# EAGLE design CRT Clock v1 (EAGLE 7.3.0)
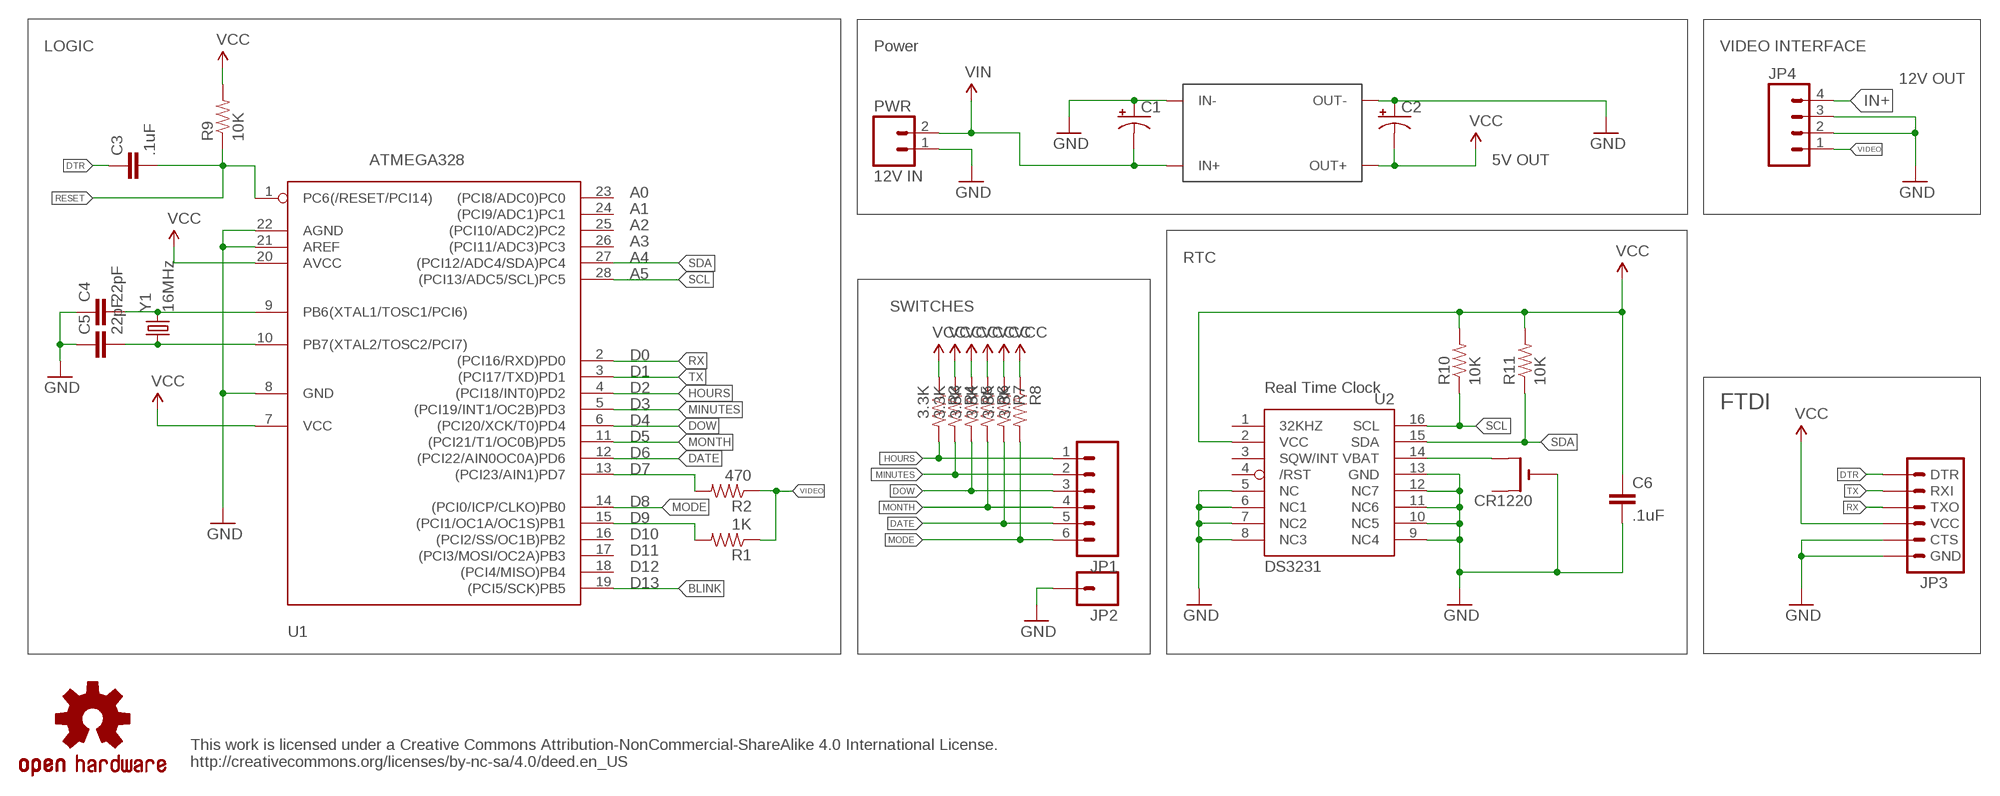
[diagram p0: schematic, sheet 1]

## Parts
C1  CAP_POLPTH2  [CPOL-RADIAL-10UF-25V]
C2  CAP_POLPTH2  [CPOL-RADIAL-10UF-25V]
C3  .1uF  CAPEZ  [CAP-PTH-SMALLEZ]
C4  22pF  CAPEZ  [CAP-PTH-SMALLEZ]
C5  22pF  CAPEZ  [CAP-PTH-SMALLEZ]
C6  .1uF  CAPEZ  [CAP-PTH-SMALLEZ]
CR1220  CR1220THM  [CR1220-THM]
JP1  M06NO_SILK_FEMALE_PTH  [1X06_NO_SILK]
JP2  M01NOSILK-KIT  [1X01NS-KIT]
JP3  ARDUINO_SERIAL_PROGRAMSMD  [1X06-SMD]
JP4  M04NO_SILK_ALL_ROUND  [1X04_NO_SILK_ALL_ROUND]
PWR  12V IN  M02PTH  [1X02]
R1  1K  RESISTORPTH-1/4W-VERT  [AXIAL-0.1]
R2  470  RESISTORPTH-1/4W-VERT  [AXIAL-0.1]
R3  3.3K  RESISTORPTH-1/4W-VERT  [AXIAL-0.1]
R4  3.3K  RESISTORPTH-1/4W-VERT  [AXIAL-0.1]
R5  3.3K  RESISTORPTH-1/4W-VERT  [AXIAL-0.1]
R6  3.3K  1KOHM-1/4W-5%(PTH)VERT  [AXIAL-0.1]
R7  3.3K  RESISTORPTH-1/4W-VERT  [AXIAL-0.1]
R8  3.3K  RESISTORPTH-1/4W-VERT  [AXIAL-0.1]
R9  10K  RESISTORPTH-1/4W-VERT  [AXIAL-0.1]
R10  10K  RESISTORPTH-1/4W-VERT  [AXIAL-0.1]
R11  10K  RESISTORPTH-1/4W-VERT  [AXIAL-0.1]
U1  ATMEGA328  ATMEGA168PROUND  [DIL28-3-ROUND]
U2  DS3231  DS3231/SO  [SO16W]
U$1  DCTODC  [DCTODC]
U$7  OSHW-LOGOS  [OSHW-LOGO-S]
Y1  16MHz  CRYSTALHC49US  [HC49US]

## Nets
BLINK: U1.19((PCI5/SCK)PB5)
DATE: JP1.5 R7.P$2 U1.12((PCI22/AIN0OC0A)PD6)
DOW: JP1.3 R5.P$2 U1.6((PCI20/XCK/T0)PD4)
DTR: C3.1 JP3.1(DTR)
GND: C1.1(+) C2.1(+) C4.1 C5.1 C6.2 CR1220.- JP2.1 JP3.5(CTS) JP3.6(GND) JP4.2 JP4.3 PWR.1 U1.8(GND) U1.21(AREF) U1.22(AGND) U2.5(NC) U2.6(NC1) U2.7(NC2) U2.8(NC3) U2.9(NC4) U2.10(NC5) U2.11(NC6) U2.12(NC7) U2.13(GND) U$1.IN- U$1.OUT-
HOURS: JP1.1 R3.P$2 U1.4((PCI18/INT0)PD2)
IN+: C1.2(-) JP4.4 PWR.2 U$1.IN+ ; supply symbol labelled VIN
MINUTES: JP1.2 R4.P$2 U1.5((PCI19/INT1/OC2B)PD3)
MODE: JP1.6 R8.P$2 U1.14((PCI0/ICP/CLKO)PB0)
MONTH: JP1.4 R6.P$2 U1.11((PCI21/T1/OC0B)PD5)
N$1: R2.P$2 U1.13((PCI23/AIN1)PD7)
N$2: CR1220.+2(+1) U2.14(VBAT)
N$3: R1.P$2 U1.15((PCI1/OC1A/OC1S)PB1)
N$37: C4.2 U1.9(PB6(XTAL1/TOSC1/PCI6)) Y1.2
N$38: C5.2 U1.10(PB7(XTAL2/TOSC2/PCI7)) Y1.1
RESET: C3.2 R9.P$1 U1.1(PC6(/RESET/PCI14))
RX: JP3.3(TXO) U1.2((PCI16/RXD)PD0)
SCL: R10.P$1 U1.28((PCI13/ADC5/SCL)PC5) U2.16(SCL)
SDA: R11.P$1 U1.27((PCI12/ADC4/SDA)PC4) U2.15(SDA)
TX: JP3.2(RXI) U1.3((PCI17/TXD)PD1)
VCC: C2.2(-) C6.1 JP3.4(VCC) R3.P$1 R4.P$1 R5.P$1 R6.P$1 R7.P$1 R8.P$1 R9.P$2 R10.P$2 R11.P$2 U1.7(VCC) U1.20(AVCC) U2.2(VCC) U$1.OUT+
VIDEO: JP4.1 R1.P$1 R2.P$1
Unconnected: CR1220.+1(+) U1.16((PCI2/SS/OC1B)PB2) U1.17((PCI3/MOSI/OC2A)PB3) U1.18((PCI4/MISO)PB4) U1.23((PCI8/ADC0)PC0) U1.24((PCI9/ADC1)PC1) U1.25((PCI10/ADC2)PC2) U1.26((PCI11/ADC3)PC3) U2.1(32KHZ) U2.3(SQW/INT) U2.4(/RST)

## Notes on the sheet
- LOGIC | Power | VIDEO INTERFACE
- 12V OUT
- 5V OUT
- A0
- A1
- A2
- A3
- A4 | RTC
- A5
- SWITCHES
- D0
- D1
- D2 | Real Time Clock
- D3 | FTDI
- D4
- D5
- D6
- D7
- D8
- D9
- D10
- D11
- D12
- D13
- This work is licensed under a Creative Commons Attribution-NonCommercial-ShareAlike 4.0 International License.
  http://creativecommons.org/licenses/by-nc-sa/4.0/deed.en_US

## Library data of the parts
C1 C2 = SparkFun-Capacitors:CAP_POL: Capacitor Polarized
C3-C6 = SparkFun-Capacitors:CAP: Capacitor
CR1220 = adafruit:CR1220: CR1216/CR1220/CR1225 12mm 3V lithium coin cell Great for battery packup. Both SMT and THM holders. Note the THM package has the ground pads on both sides of the PCB so that the masks are the same - this reduces the cost
JP1 = SparkFun-Connectors:M06: Header 6 Standard 6-pin 0.1" header. Use with straight break away headers (SKU : PRT-00116), right angle break away headers (PRT-00553), swiss pins (PRT-00743), machine pins (PRT-00117), and female headers (PRT-00115). Molex polarized connector foot print use with SKU : PRT-08094 with associated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; PROD_ID: CONN-08437
JP2 = SparkFun-Connectors:M01: Header 1
JP3 = SparkFun-Connectors:ARDUINO_SERIAL_PROGRAM: FTDI connector footprints; PROD_ID: CONN-08971
JP4 = SparkFun-Connectors:M04: Header 4 Standard 4-pin 0.1" header. Use with straight break away headers (SKU : PRT-00116), right angle break away headers (PRT-00553), swiss pins (PRT-00743), machine pins (PRT-00117), and female headers (PRT-00115). Molex polarized connector foot print use with SKU : PRT-08231 with associated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
PWR = SparkFun w:epaper:M02: Header 2
R1-R5 R7-R11 = SparkFun-Resistors:RESISTOR: Resistor
R6 = SparkFun-Resistors:1KOHM-1/4W-5%(PTH): RES-08380; PROD_ID: RES-08380; VALUE: 1k
U1 = adafruit:ATMEGA168*P: MICROCONTROLLER 16 kBytes FLASH 1 kBytes SRAM 512 Bytes EEPROM USART 8-channel 10 bit ADC
U2 = adafruit:DS3231
U$1 = DC to DC:DCTODC
U$7 = SparkFun:OSHW-LOGO: Open Source Hardware Logo This logo indicates the piece of hardware it is found on incorporates a OSHW license and/or adheres to the definition of open source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
Y1 = SparkFun-FreqCtrl:CRYSTAL: Various standard crystals. Proven footprints.

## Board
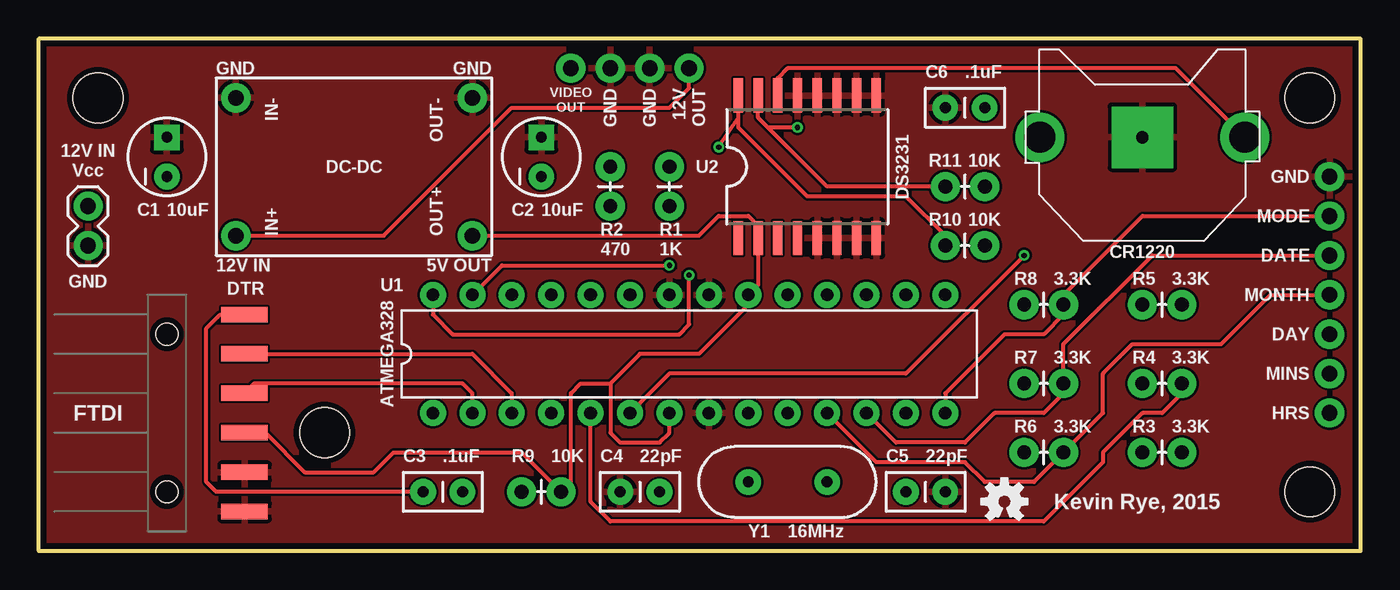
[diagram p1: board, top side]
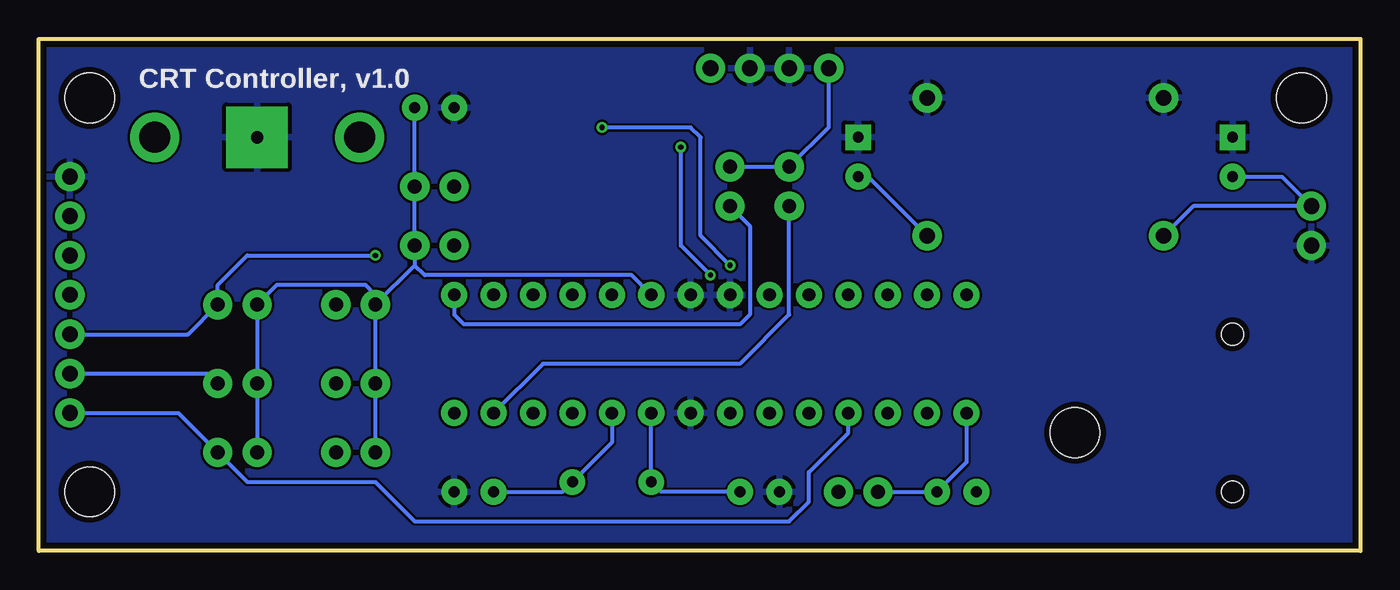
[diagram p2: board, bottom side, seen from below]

Size 85.19 x 33.02 mm. Coordinates in mm from the lower left corner, seen from the top.
Outline: 0,0 85.19,0 85.19,33.02 0,33.02 0,0
Copper layers (1*16): Top 0.0356mm / dielectric 1.5011mm / Bottom 0.0356mm
Design rules "LaenPCBOrder": minimum track width 6mil, minimum drill 13mil, track to track 6mil, track to pad 6mil, pad to pad 6mil, via to via 6mil, smd to smd 6mil, copper to edge 15mil, drill to drill 6mil, minimum pad ring 7mil, minimum via ring 7mil, stop-mask expansion 3mil, vias tented up to drill 0mil, thermal gap 10mil
Holes 3.2 mm at 81.92,3.81 81.92,29.21 3.81,29.21 18.42,7.62

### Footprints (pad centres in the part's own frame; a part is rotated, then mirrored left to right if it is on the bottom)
CPOL-RADIAL-10UF-25V = drill 0.7 pad 1.651 square: 1 1.27,0 | drill 0.7 pad 1.651: 2 -1.27,0
CAP-PTH-SMALLEZ = drill 0.7 pad 1.651: 1 0,0; 2 2.54,0
CR1220-THM = drill 2 pad 3.175: +1 -6.604,0; +2 6.604,0 | drill 0.8 pad 3.962 square: - 0,0
1X06_NO_SILK = drill 1.016 pad 1.88: 1 0,0; 2 2.54,0; 3 5.08,0; 4 7.62,0; 5 10.16,0; 6 12.7,0
1X01NS-KIT = drill 1.016 pad 1.88: 1 0,0
1X06-SMD = smd 1 x 3: 1 -6.35,5; 2 -3.81,5; 3 -1.27,5; 4 1.27,5; 5 3.81,5; 6 6.35,5 | hole 1.4: -5.08,0; 5.08,0
1X04_NO_SILK_ALL_ROUND = drill 1.016 pad 1.88: 1 0,0; 2 2.54,0; 3 5.08,0; 4 7.62,0
1X02 = drill 1.016 pad 1.88: 1 0,0; 2 2.54,0
AXIAL-0.1 = drill 0.9 pad 1.88: P$1 0,0; P$2 2.54,0
DIL28-3-ROUND = drill 0.813 pad 1.676: 1 -16.51,-3.81; 2 -13.97,-3.81; 3 -11.43,-3.81; 4 -8.89,-3.81; 5 -6.35,-3.81; 6 -3.81,-3.81; 7 -1.27,-3.81; 8 1.27,-3.81; 9 3.81,-3.81; 10 6.35,-3.81; 11 8.89,-3.81; 12 11.43,-3.81; 13 13.97,-3.81; 14 16.51,-3.81; 15 16.51,3.81; 16 13.97,3.81; 17 11.43,3.81; 18 8.89,3.81; 19 6.35,3.81; 20 3.81,3.81; 21 1.27,3.81; 22 -1.27,3.81; 23 -3.81,3.81; 24 -6.35,3.81; 25 -8.89,3.81; 26 -11.43,3.81; 27 -13.97,3.81; 28 -16.51,3.81
SO16W = smd 0.6 x 2.2: 1 -4.445,-4.6; 2 -3.175,-4.6; 3 -1.905,-4.6; 4 -0.635,-4.6; 5 0.635,-4.6; 6 1.905,-4.6; 7 3.175,-4.6; 8 4.445,-4.6; 9 4.445,4.6; 10 3.175,4.6; 11 1.905,4.6; 12 0.635,4.6; 13 -0.635,4.6; 14 -1.905,4.6; 15 -3.175,4.6; 16 -4.445,4.6
DCTODC = drill 1.016 pad 1.88: IN+ 10.16,1.27; IN- 1.27,1.27; OUT+ 10.16,16.51; OUT- 1.27,16.51
HC49US = drill 0.7 pad 1.651: 1 -2.54,0; 2 2.54,0

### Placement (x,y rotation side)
C1  8.26,25.4 90 top
C2  32.38,25.4 90 top
C3  24.77,3.81 0 top
C4  37.46,3.81 0 top
C5  58.42,3.81 180 top
C6  60.96,28.58 180 top
CR1220  71.12,26.67 0 top
JP1  83.19,8.89 90 top
JP2  83.19,24.13 90 top
JP3  8.26,8.89 270 top
JP4  34.29,31.12 0 top
PWR  3.17,19.69 90 top
R1  40.64,24.77 270 top
R2  36.83,24.77 270 top
R3  71.12,6.35 0 top
R4  71.12,10.79 0 top
R5  71.12,15.88 0 top
R6  63.5,6.35 0 top
R7  63.5,10.79 0 top
R8  63.5,15.88 0 top
R9  31.12,3.81 0 top
R10  58.42,19.69 0 top
R11  58.42,23.5 0 top
U1  41.91,12.7 0 top
U2  49.53,24.77 0 top
U$1  11.43,30.48 270 top
U$7  62.23,3.17 0 top
Y1  48.26,4.45 180 top

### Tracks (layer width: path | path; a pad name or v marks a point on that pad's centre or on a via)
DATE
  Top 0.254: JP1.5 71.76,19.05 66.04,13.33 R7.P$2 66.04,10.16 64.77,8.89 61.59,8.89 59.69,6.98 55.24,6.98 U1.12
DOW  (via drill 0.33 pad 0.69)
  Top 0.254: v63.5,19.05 55.88,11.43 40.64,11.43 U1.6
  Bottom 0.254: JP1.3 75.57,13.97 R5.P$2 73.66,17.15 71.76,19.05 v63.5,19.05
DTR
  Top 0.254: C3.1 11.43,3.81 10.79,4.45 10.79,14.34 11.69,15.24 JP3.1
GND
  pour Top: -1.27,34.29 86.36,34.29 86.36,-1.27 -1.27,-1.27
  pour Bottom: -0.64,33.66 85.73,33.66 85.73,-0.64 -0.64,-0.64
HOURS
  Bottom 0.254: JP1.1 76.2,8.89 R3.P$2 71.76,4.45 63.5,4.45 60.96,1.91 36.83,1.91 35.56,3.17 35.56,5.08 33.02,7.62 U1.4
IN+
  Top 0.254: U$1.IN+ 22.23,20.32 30.48,28.58 40.64,28.58 41.91,29.85 JP4.4
  Bottom 0.254: U$1.IN+ 10.79,22.23 PWR.2 5.08,24.13 C1.2
MINUTES
  Top 0.254: R4.P$2 73.66,10.16 72.39,8.89 71.12,8.89 68.58,6.35 68.58,5.71 64.77,1.91 36.83,1.91 35.56,3.17 U1.5
  Bottom 0.254: JP1.2 74.3,11.43 R4.P$2
MODE
  Top 0.254: JP1.6 71.12,21.59 66.04,16.51 R8.P$2 66.04,15.24 64.77,13.97 62.23,13.97 58.42,10.16 U1.14
MONTH
  Top 0.254: U1.11 53.98,5.71 59.69,5.71 60.96,4.45 64.14,4.45 R6.P$2 68.58,8.89 68.58,11.43 70.48,13.33 76.2,13.33 79.38,16.51 JP1.4
N$1
  Bottom 0.254: U1.13 52.7,12.06 40,12.06 36.83,15.24 R2.P$2
N$2
  Top 0.254: CR1220.+2 73.28,31.12 48.26,31.12 47.62,30.48 U2.14
N$3
  Bottom 0.254: U1.15 58.42,15.24 57.78,14.61 40,14.61 39.37,15.24 39.37,20.96 R1.P$2
N$37
  Bottom 0.254: C4.2 45.09,3.81 Y1.2 U1.9
N$38
  Bottom 0.254: C5.2 51.43,3.81 Y1.1 48.26,6.98 U1.10
RESET
  Bottom 0.254: R9.P$1 C3.2 25.4,5.71 U1.1
RX
  Top 0.254: U1.2 27.94,10.16 27.31,10.79 13.89,10.79 JP3.3
SCL  (via drill 0.33 pad 0.69)
  Top 0.254: R10.P$1 58.42,20.32 55.88,22.86 49.53,22.86 45.09,27.31 45.09,27.94 | 45.09,27.94 U2.16 | U1.28 25.4,15.24 26.67,13.97 41.27,13.97 41.91,14.61 v41.91,17.78 | v43.81,26.04 45.09,27.94
  Bottom 0.254: v41.91,17.78 43.81,19.69 v43.81,26.04
SDA  (via drill 0.33 pad 0.69)
  Top 0.254: R11.P$1 50.8,23.5 46.99,27.31 | 46.99,27.31 46.35,27.94 U2.15 | U1.27 29.85,18.42 v40.64,18.42 | v48.89,27.31 46.99,27.31
  Bottom 0.254: v40.64,18.42 42.54,20.32 42.54,26.67 43.18,27.31 v48.89,27.31
TX
  Top 0.254: JP3.2 27.94,12.7 30.48,10.16 U1.3
VCC
  Top 0.254: U$1.OUT+ 42.54,20.32 43.81,21.59 45.72,21.59 46.35,20.96 U2.2 46.35,17.15 U1.20 45.72,15.88 42.54,12.7 38.73,12.7 36.83,10.79 | 36.83,10.79 36.83,7.62 37.46,6.98 40,6.98 40.64,7.62 U1.7 | 36.83,10.79 34.92,10.79 34.29,10.16 34.29,4.45 R9.P$2 31.12,6.35 22.86,6.35 21.59,5.08 17.15,5.08 14.61,7.62 JP3.4
  Bottom 0.254: C6.1 R11.P$2 R10.P$2 60.96,18.42 | 60.96,18.42 R8.P$1 | R8.P$1 R7.P$1 R6.P$1 | R8.P$1 63.5,16.51 64.14,17.15 69.85,17.15 R5.P$1 R4.P$1 R3.P$1 | U1.20 46.99,17.78 60.32,17.78 60.96,18.42 | C2.2 31.75,24.13 U$1.OUT+
VIDEO
  Bottom 0.254: R1.P$1 R2.P$1 34.29,27.31 JP4.1

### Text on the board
Unrouted: This work is licensed under a Creative Commons Attribution-NonCommercial-ShareAlike 4.0 International License. / http://creativecommons.org/licenses/by-nc-sa/4.0/deed.en_US
tPlace: GND | GND | VIDEO | GND | GND | 12V | OUT | OUT | 12V IN | DC-DC | Vcc | GND | 10uF | 10uF | MODE | 12V IN | 5V OUT | DATE | GND | DTR | MONTH | DAY | MINS | FTDI | HRS | Kevin Rye, 2015
bPlace: CRT Controller, v1.0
